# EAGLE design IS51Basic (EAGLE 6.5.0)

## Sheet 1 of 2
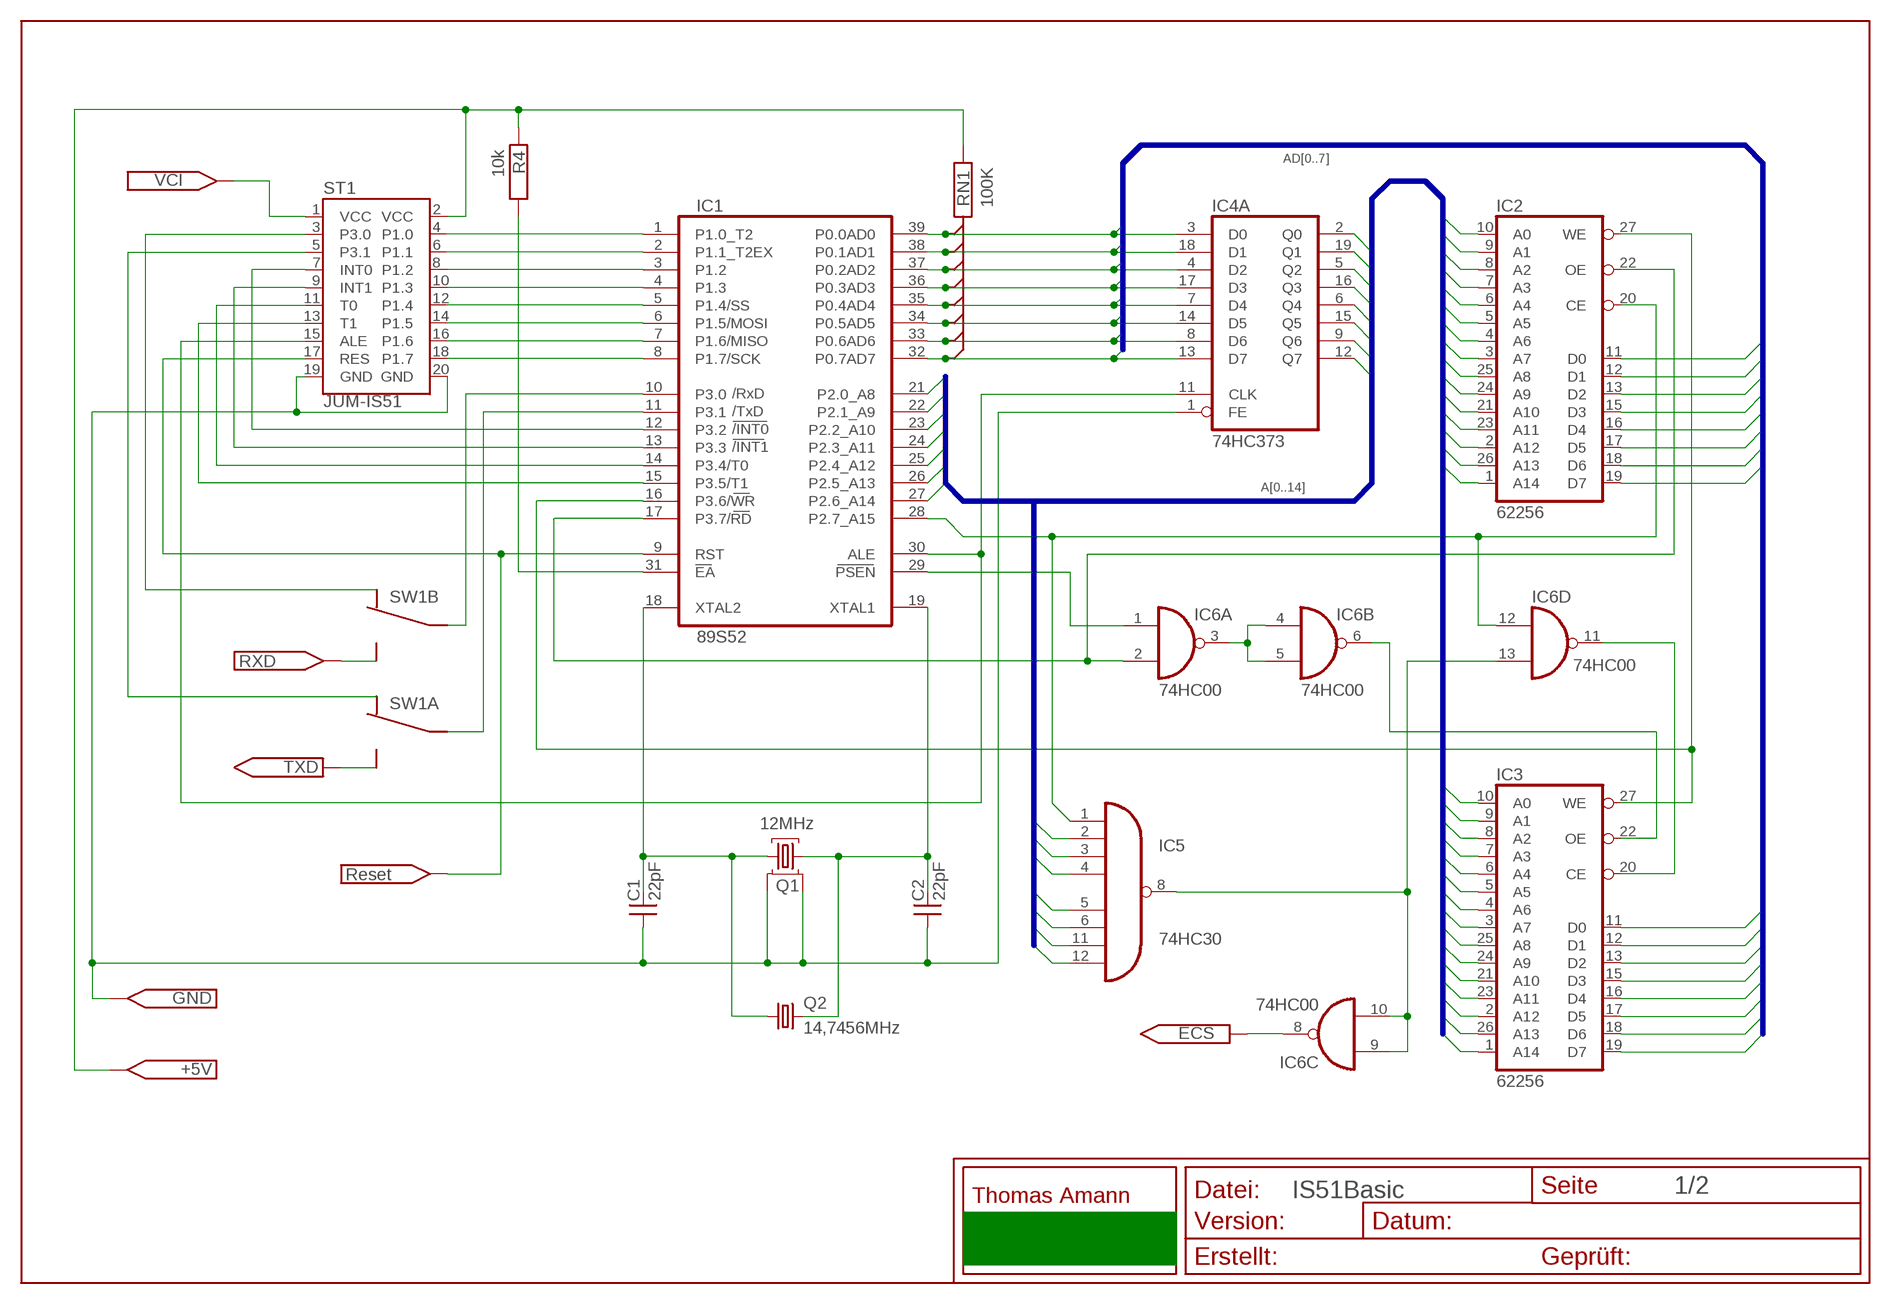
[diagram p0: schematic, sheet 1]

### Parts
C1  22pF  C2_025  [C2_025]
C2  22pF  C2_025  [C2_025]
IC1  89S52  89S8253  [DIL40]
IC2  62256  62256DIL28_SMAL  [DIL28_S]
IC3  62256  [DIL28]
IC4  74HC373  74373_1  [DIL20]
IC5  74HC30  74HC30N  [DIL14]
IC6  74HC00  74HC00N  [DIL14]
Q1  12MHz  QUARZ4  [QCTS406]
Q2  14,7456MHz  CRYSTALHC49S  [HC49/S]
R4  10k  R025A  [R025A]
RN1  100K  RN8_DIL  [RN8_DIL]
ST1  JUM-IS51  [JUM10X2]
SW1  SW2_2XUM  [SW2_2XUM]

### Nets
A0: IC2.10(A0) IC3.10(A0) IC4.2(A:Q0) ; also sheet 2
A1: IC2.9(A1) IC3.9(A1) IC4.19(A:Q1) ; also sheet 2
A2: IC2.8(A2) IC3.8(A2) IC4.5(A:Q2) ; also sheet 2
A3: IC2.7(A3) IC3.7(A3) IC4.16(A:Q3) ; also sheet 2
A4: IC2.6(A4) IC3.6(A4) IC4.6(A:Q4) ; also sheet 2
A5: IC2.5(A5) IC3.5(A5) IC4.15(A:Q5) ; also sheet 2
A6: IC2.4(A6) IC3.4(A6) IC4.9(A:Q6) ; also sheet 2
A7: IC2.3(A7) IC3.3(A7) IC4.12(A:Q7) ; also sheet 2
A8: IC1.21(P2.0_A8) IC2.25(A8) IC3.25(A8) IC5.11(I6) ; also sheet 2
A9: IC1.22(P2.1_A9) IC2.24(A9) IC3.24(A9) IC5.12(I7) ; also sheet 2
A10: IC1.23(P2.2_A10) IC2.21(A10) IC3.21(A10) IC5.6(I5) ; also sheet 2
A11: IC1.24(P2.3_A11) IC2.23(A11) IC3.23(A11) IC5.5(I4) ; also sheet 2
A12: IC1.25(P2.4_A12) IC2.2(A12) IC3.2(A12) IC5.4(I3) ; also sheet 2
A13: IC1.26(P2.5_A13) IC2.26(A13) IC3.26(A13) IC5.3(I2) ; also sheet 2
A14: IC1.27(P2.6_A14) IC2.1(A14) IC3.1(A14) IC5.2(I1) ; also sheet 2
A15: IC1.28(P2.7_A15) IC2.20(CE) IC5.1(I0) IC6.12(D:I0) ; also sheet 2
AD0: IC1.39(P0.0AD0) IC2.11(D0) IC3.11(D0) IC4.3(A:D0) RN1.2 ; also sheet 2
AD1: IC1.38(P0.1AD1) IC2.12(D1) IC3.12(D1) IC4.18(A:D1) RN1.3 ; also sheet 2
AD2: IC1.37(P0.2AD2) IC2.13(D2) IC3.13(D2) IC4.4(A:D2) RN1.4 ; also sheet 2
AD3: IC1.36(P0.3AD3) IC2.15(D3) IC3.15(D3) IC4.17(A:D3) RN1.5 ; also sheet 2
AD4: IC1.35(P0.4AD4) IC2.16(D4) IC3.16(D4) IC4.7(A:D4) RN1.6 ; also sheet 2
AD5: IC1.34(P0.5AD5) IC2.17(D5) IC3.17(D5) IC4.14(A:D5) RN1.7 ; also sheet 2
AD6: IC1.33(P0.6AD6) IC2.18(D6) IC3.18(D6) IC4.8(A:D6) RN1.8 ; also sheet 2
AD7: IC1.32(P0.7AD7) IC2.19(D7) IC3.19(D7) IC4.13(A:D7) RN1.9 ; also sheet 2
ALE: IC1.30(ALE) IC4.11(A:CLK) ST1.15(ALE)
EA: IC1.31(EA) R4.2
ECS: IC6.8(C:O) ; also sheet 2
GND: C1.1 C2.1 IC4.1(A:FE) Q1.2 Q1.4 ST1.19(GND) ST1.20(GND) ; also sheet 2
INT0: IC1.12(P3.2) ST1.7(INT0)
INT1: IC1.13(P3.3) ST1.9(INT1)
N$14: IC3.20(CE) IC6.11(D:O)
N$15: IC5.8(O) IC6.9(C:I0) IC6.10(C:I1) IC6.13(D:I1)
OER: IC3.22(OE) IC6.6(B:O)
OEV: IC6.3(A:O) IC6.4(B:I0) IC6.5(B:I1)
P10: IC1.1(P1.0_T2) ST1.4(P1.0)
P11: IC1.2(P1.1_T2EX) ST1.6(P1.1)
P12: IC1.3(P1.2) ST1.8(P1.2)
P13: IC1.4(P1.3) ST1.10(P1.3)
P14: IC1.5(P1.4/SS) ST1.12(P1.4)
P15: IC1.6(P1.5/MOSI) ST1.14(P1.5)
P16: IC1.7(P1.6/MISO) ST1.16(P1.6)
P17: IC1.8(P1.7/SCK) ST1.18(P1.7)
P30: ST1.3(P3.0) SW1.6
P31: ST1.5(P3.1) SW1.1
PSEN: IC1.29(PSEN) IC6.1(A:I0)
RD: IC1.17(P3.7/RD) IC2.22(OE) IC6.2(A:I1) ; also sheet 2
RES: IC1.9(RST) ST1.17(RES) ; also sheet 2
RXP: IC1.10(P3.0) SW1.5
T0: IC1.14(P3.4/T0) ST1.11(T0)
T1: IC1.15(P3.5/T1) ST1.13(T1)
TXD: SW1.3 ; also sheet 2
TXP: IC1.11(P3.1) SW1.2
VCC: R4.1 RN1.1 ST1.2(VCC) ; also sheet 2
VCI: ST1.1(VCC) ; also sheet 2
WR: IC1.16(P3.6/WR) IC2.27(WE) IC3.27(WE) ; also sheet 2
XT1: C2.2 IC1.19(XTAL1) Q1.3 Q2.2
XT2: C1.2 IC1.18(XTAL2) Q1.1 Q2.1
XYZ: SW1.4 ; also sheet 2

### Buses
A[0..14]
AD[0..7]

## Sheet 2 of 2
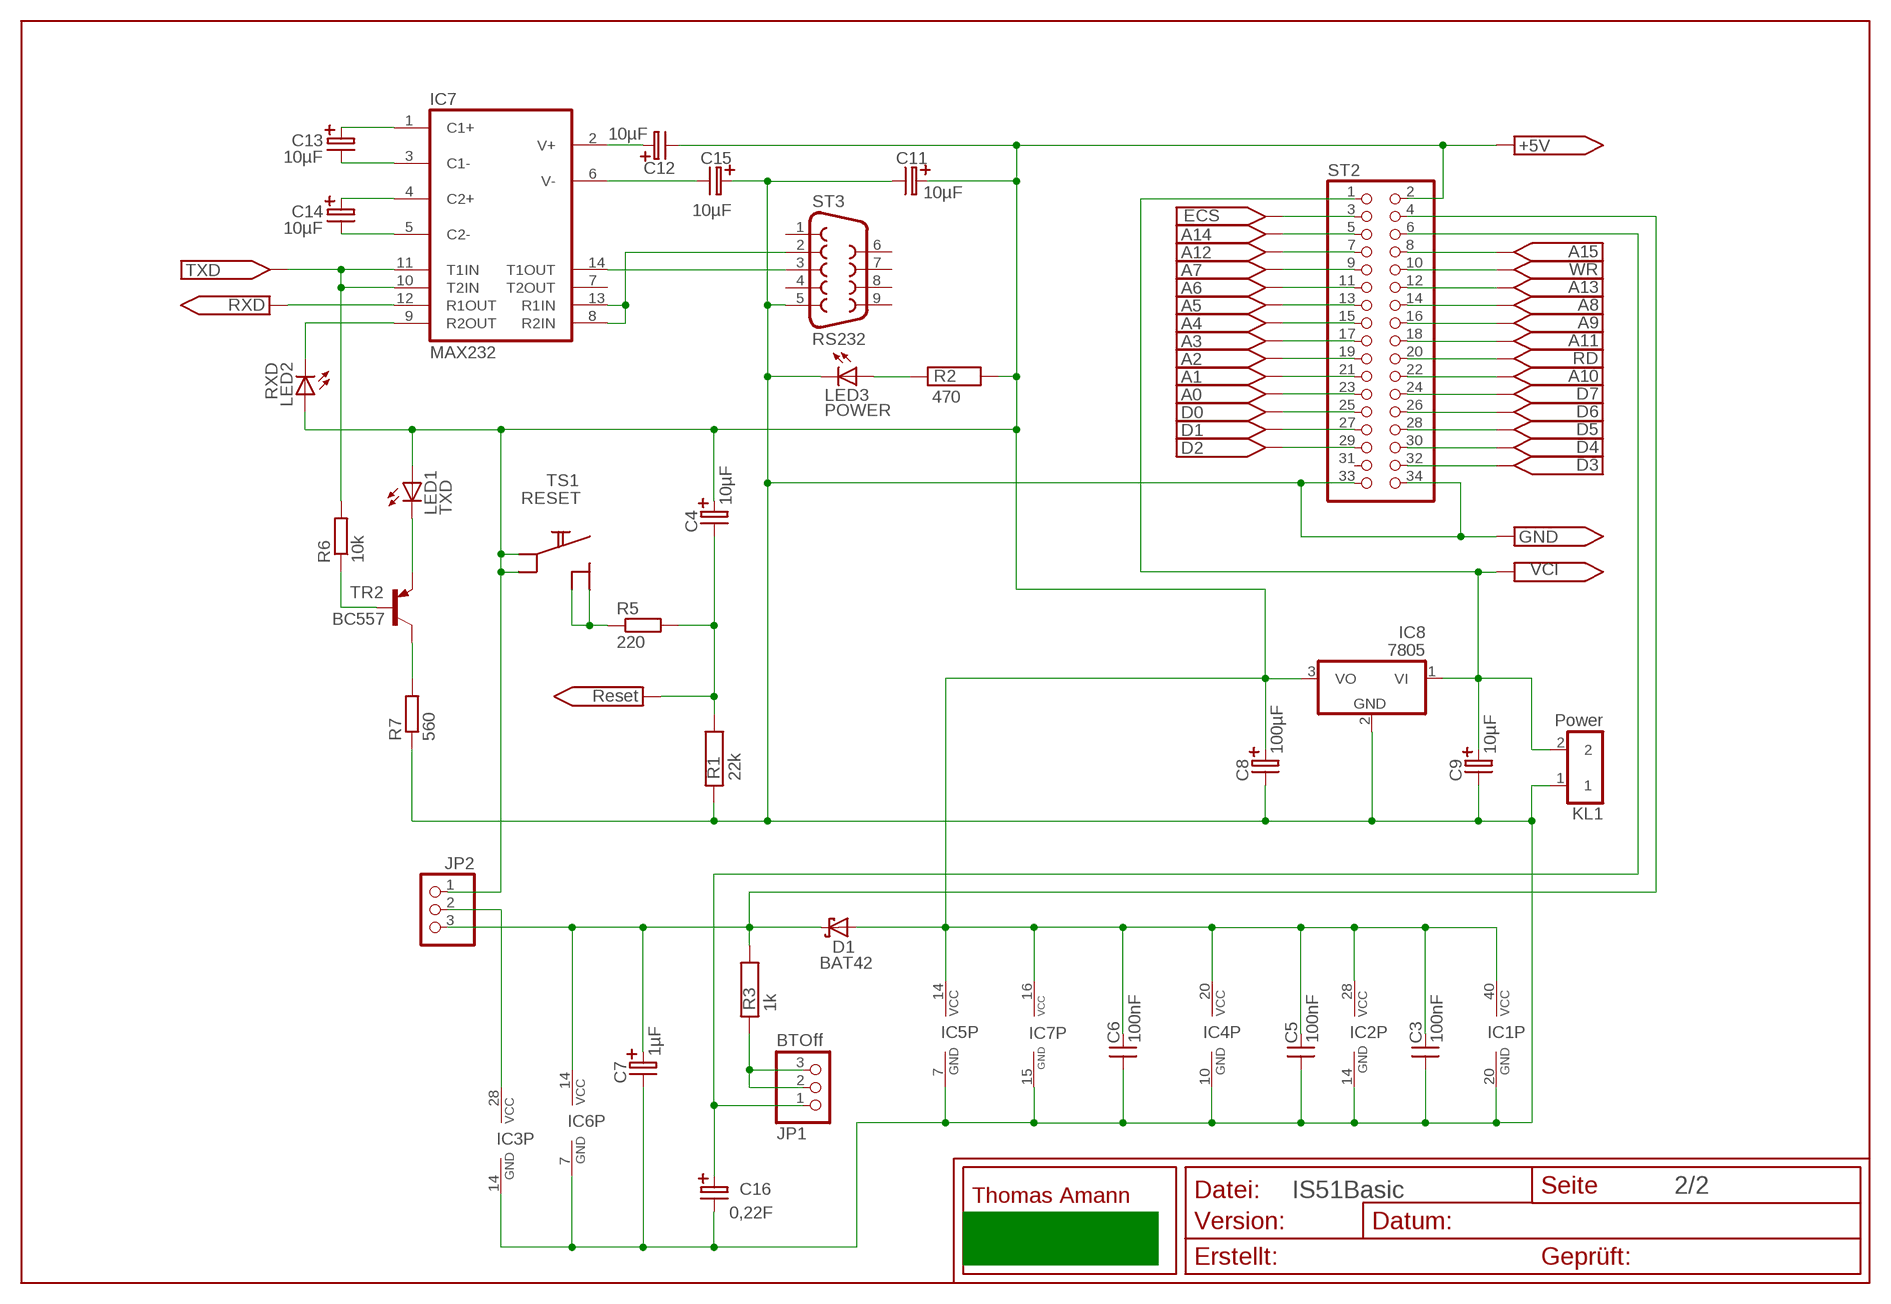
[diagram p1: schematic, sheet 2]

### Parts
C3  100nF  C2_05  [C2_05]
C4  10µF  TELK1_25  [TELK1_25]
C5  100nF  C2_05  [C2_05]
C6  100nF  C2_05  [C2_05]
C7  1µF  TELK1_25  [TELK1_25]
C8  100µF  TELK1_25  [TELK1_25]
C9  10µF  TELK1_25  [TELK1_25]
C11  10µF  TELK1_25  [TELK1_25]
C12  10µF  TELK1_25  [TELK1_25]
C13  10µF  TELK1_25  [TELK1_25]
C14  10µF  TELK1_25  [TELK1_25]
C15  10µF  TELK1_25  [TELK1_25]
C16  0,22F  E50_125R  [E50_125R]
D1  BAT42  [DO35-10]
IC7  MAX232  [DIL16]
IC8  7805  7805TV  [TO220V]
JP1  BTOff  PINHD-1X3  [1X03]
JP2  PINHD-1X3  [1X03]
KL1  Power  KL2_5  [KL2_5]
LED1  TXD  LED3MM  [LED3MM]
LED2  RXD  LED3MM  [LED3MM]
LED3  POWER  LED3MM  [LED3MM]
R1  22k  R025A  [R025A]
R2  470  R025A  [R025A]
R3  1k  R025A  [R025A]
R5  220  R-EU_R1206  [R1206]
R6  10k  R-EU_R1206  [R1206]
R7  560  R-EU_R1206  [R1206]
ST2  PINHD-2X17  [2X17]
ST3  RS232  F09H  [F09H]
TR2  BC557  BC327  [TO92]
TS1  RESET  MTAST  [MTAST]

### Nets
A0: ST2.23 ; also sheet 1
A1: ST2.21 ; also sheet 1
A2: ST2.19 ; also sheet 1
A3: ST2.17 ; also sheet 1
A4: ST2.15 ; also sheet 1
A5: ST2.13 ; also sheet 1
A6: ST2.11 ; also sheet 1
A7: ST2.9 ; also sheet 1
A8: ST2.14 ; also sheet 1
A9: ST2.16 ; also sheet 1
A10: ST2.22 ; also sheet 1
A11: ST2.18 ; also sheet 1
A12: ST2.7 ; also sheet 1
A13: ST2.12 ; also sheet 1
A14: ST2.5 ; also sheet 1
A15: ST2.8 ; also sheet 1
AD0: ST2.25 ; also sheet 1
AD1: ST2.27 ; also sheet 1
AD2: ST2.29 ; also sheet 1
AD3: ST2.32 ; also sheet 1
AD4: ST2.30 ; also sheet 1
AD5: ST2.28 ; also sheet 1
AD6: ST2.26 ; also sheet 1
AD7: ST2.24 ; also sheet 1
ECS: ST2.3 ; also sheet 1
GND: C3.1 C5.1 C6.1 C7.K C8.K C9.K C11.K C15.A C16.K IC1.20(GND) IC2.14(GND) IC3.14(GND) IC4.10(P:GND) IC5.7(GND) IC6.7(P:GND) IC7.15(GND) IC8.2(GND) KL1.1 LED3.K(C) R1.1 R7.1 ST2.33 ST2.34 ST3.5 ; also sheet 1
N$1: C13.K IC7.3(C1-)
N$4: C13.A IC7.1(C1+)
N$6: LED3.A R2.1
N$13: LED1.K(C) TR2.1(E)
N$18: C14.A IC7.4(C2+)
N$19: C14.K IC7.5(C2-)
N$23: R6.1 TR2.2(B)
N$25: R7.2 TR2.3(C)
N$28: IC7.14(T1OUT) ST3.3
N$29: IC7.8(R2IN) IC7.13(R1IN) ST3.2
N$31: C15.K IC7.6(V-)
N$32: C12.A IC7.2(V+)
N$49: R5.1 TS1.3 TS1.4
RD: ST2.20 ; also sheet 1
RES: C4.K R1.2 R5.2 ; also sheet 1
RXL: IC7.9(R2OUT) LED2.K(C)
TXD: IC7.10(T2IN) IC7.11(T1IN) R6.2 ; also sheet 1
VCB: C16.A JP1.1 ST2.6
VCC: C3.2 C4.A C5.2 C6.2 C8.A C11.A C12.K D1.A IC1.40(VCC) IC2.28(VCC) IC4.20(P:VCC) IC5.14(VCC) IC7.16(VCC) IC8.3(VO) JP2.1 LED1.A LED2.A R2.2 ST2.2 TS1.1 TS1.2 ; also sheet 1
VCI: C9.A IC8.1(VI) KL1.2 ST2.1 ; also sheet 1
VCP: C7.A D1.C IC6.14(P:VCC) JP2.3 R3.2 ST2.4
VCR: IC3.28(VCC) JP2.2
VCV: JP1.2 JP1.3 R3.1
WR: ST2.10 ; also sheet 1
XYZ: IC7.12(R1OUT) ; also sheet 1
Unconnected: IC7.7(T2OUT) ST2.31 ST3.1 ST3.4 ST3.6 ST3.7 ST3.8 ST3.9

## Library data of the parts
C1 C2 = RUNDC:C2_025
C3 C5 C6 = RUNDC:C2_05
C4 C7-C9 C11-C15 = RUNDC:TELK1_25
C16 = RUNDC:E50_125R
D1 = diode:BAT42: DIODE
IC1 = IS-51:89S8253: Grundmodel 8051/32 in DIL40 und PLCC44
IC2 = MyMemory:62256: Static-RAM 32k x 8
IC3 = memory:62256
IC4 = IS-51:74373_1: 74373 mit D0-D7 Belegung von oben nach unten
IC5 = 74xx-eu:74*30: 8-input NAND gate
IC6 = 74xx-eu:74*00: Quad 2-input NAND gate
IC7 = maxim:MAX232: RS232 TRANSEIVER
IC8 = linear:78*: Positive VOLTAGE REGULATOR Source: http://cache.national.com/ds/LM/LM78L05.pdf http://www.fairchildsemi.com/ds/LM/LM7805.pdf
JP1 JP2 = pinhead:PINHD-1X3: PIN HEADER
KL1 = TOMLIB:KL2_5
LED1-LED3 = led:LED: LED
Q1 = TOMLIB:QUARZ4
Q2 = crystal:CRYSTAL: CRYSTAL
R1-R4 = RUNDC:R025A
R5-R7 = resistor:R-EU_: RESISTOR, European symbol
RN1 = RUNDC:RN8_DIL
ST1 = IS-51:JUM-IS51: 20pol. Stecker für Erweiterung der IS51
ST2 = pinhead:PINHD-2X17: PIN HEADER
ST3 = con-subd:F09: SUB-D
SW1 = TOMLIB:SW2_2XUM
TR2 = transistor-pnp:BC327: PNP Transistor
TS1 = TOMLIB:MTAST: Einfacher Taster mit zwei paralellen Kontakten

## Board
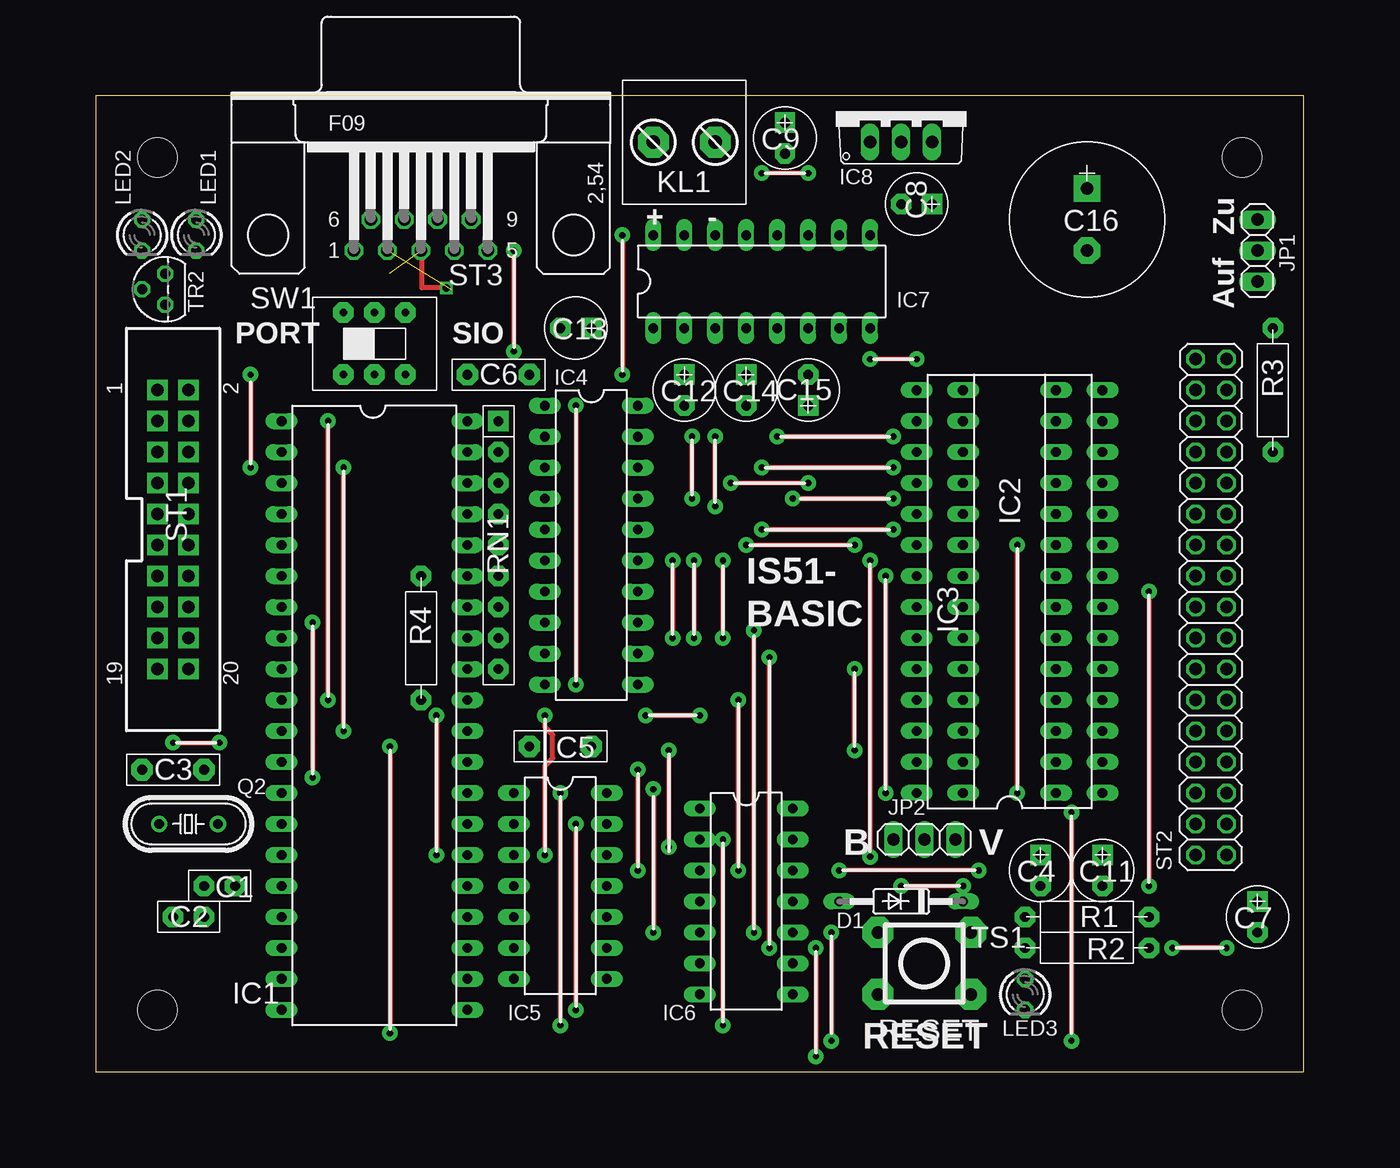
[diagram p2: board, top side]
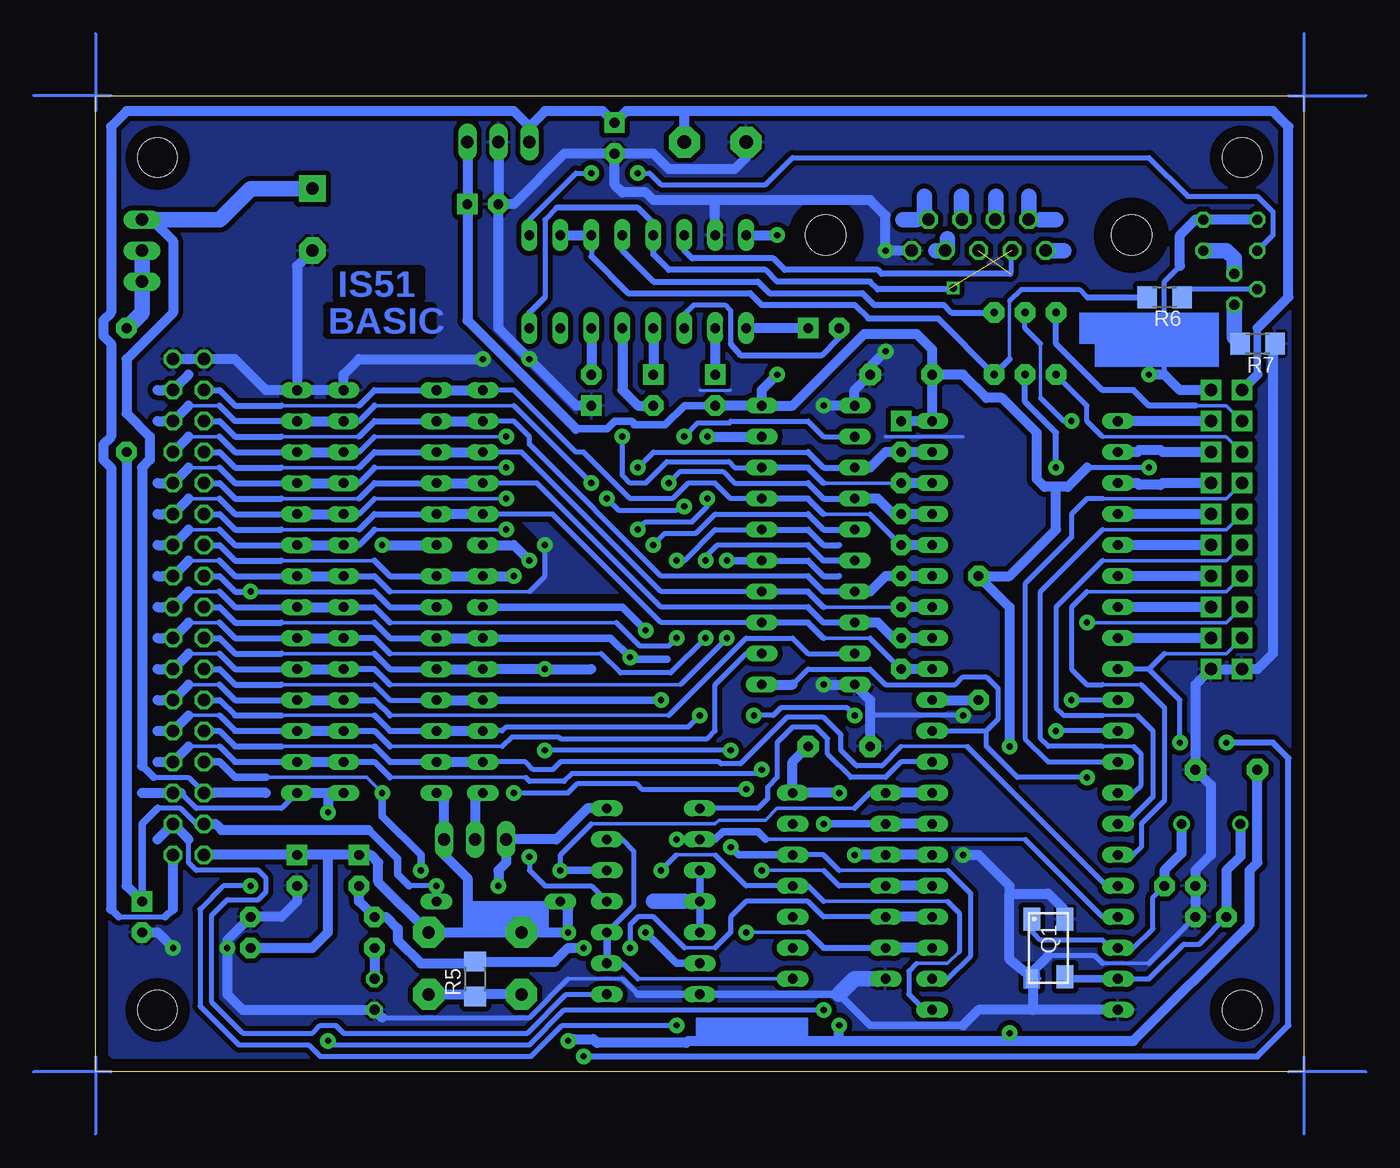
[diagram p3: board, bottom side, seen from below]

Size 99.04 x 80 mm. Coordinates in mm from the lower left corner, seen from the top.
Outline: 0,0 99.04,0 99.04,80 0,80 0,0
Copper layers (1*16): Top 0.035mm / dielectric 1.5mm / Bottom 0.035mm
Design rules "default": minimum track width 10mil, minimum drill 24mil, track to track 8mil, track to pad 8mil, pad to pad 8mil, via to via 8mil, smd to smd 8mil, copper to edge 40mil, drill to drill 8mil, minimum pad ring 10mil, minimum via ring 8mil, stop-mask expansion 4mil, vias tented up to drill 0mil, thermal gap 10mil
Holes 3.2 mm at 5.08,74.93 5.08,5.08 93.98,5.08 93.98,74.93

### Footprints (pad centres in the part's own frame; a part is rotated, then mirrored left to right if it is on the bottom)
C2_025 = drill 0.813 pad 1.676 octagon: 1 -1.27,0; 2 1.27,0
C2_05 = drill 0.813 pad 1.778 octagon: 1 0,0; 2 5.08,0
TELK1_25 = drill 0.813 pad 1.676 square: A 0,0 | drill 0.813 pad 1.676 octagon: K 0,-2.54
E50_125R = drill 1.016 pad 2.184 square: A 0,0 | drill 1.016 pad 2.184 octagon: K 0,-5.08
DO35-10 = drill 0.813 long: A 5.08,0; C -5.08,0
DIL40 = drill 0.813 long: 1 -24.13,-7.62; 2 -21.59,-7.62; 3 -19.05,-7.62; 4 -16.51,-7.62; 5 -13.97,-7.62; 6 -11.43,-7.62; 7 -8.89,-7.62; 8 -6.35,-7.62; 9 -3.81,-7.62; 10 -1.27,-7.62; 11 1.27,-7.62; 12 3.81,-7.62; 13 6.35,-7.62; 14 8.89,-7.62; 15 11.43,-7.62; 16 13.97,-7.62; 17 16.51,-7.62; 18 19.05,-7.62; 19 21.59,-7.62; 20 24.13,-7.62; 21 24.13,7.62; 22 21.59,7.62; 23 19.05,7.62; 24 16.51,7.62; 25 13.97,7.62; 26 11.43,7.62; 27 8.89,7.62; 28 6.35,7.62; 29 3.81,7.62; 30 1.27,7.62; 31 -1.27,7.62; 32 -3.81,7.62; 33 -6.35,7.62; 34 -8.89,7.62; 35 -11.43,7.62; 36 -13.97,7.62; 37 -16.51,7.62; 38 -19.05,7.62; 39 -21.59,7.62; 40 -24.13,7.62; 41 -24.13,-7.62
DIL28_S = drill 0.813 long: 1 -16.51,-3.81; 2 -13.97,-3.81; 3 -11.43,-3.81; 4 -8.89,-3.81; 5 -6.35,-3.81; 6 -3.81,-3.81; 7 -1.27,-3.81; 8 1.27,-3.81; 9 3.81,-3.81; 10 6.35,-3.81; 11 8.89,-3.81; 12 11.43,-3.81; 13 13.97,-3.81; 14 16.51,-3.81; 15 16.51,3.81; 16 13.97,3.81; 17 11.43,3.81; 18 8.89,3.81; 19 6.35,3.81; 20 3.81,3.81; 21 1.27,3.81; 22 -1.27,3.81; 23 -3.81,3.81; 24 -6.35,3.81; 25 -8.89,3.81; 26 -11.43,3.81; 27 -13.97,3.81; 28 -16.51,3.81
DIL28 = drill 0.813 long: 1 -16.51,-7.62; 2 -13.97,-7.62; 3 -11.43,-7.62; 4 -8.89,-7.62; 5 -6.35,-7.62; 6 -3.81,-7.62; 7 -1.27,-7.62; 8 1.27,-7.62; 9 3.81,-7.62; 10 6.35,-7.62; 11 8.89,-7.62; 12 11.43,-7.62; 13 13.97,-7.62; 14 16.51,-7.62; 15 16.51,7.62; 16 13.97,7.62; 17 11.43,7.62; 18 8.89,7.62; 19 6.35,7.62; 20 3.81,7.62; 21 1.27,7.62; 22 -1.27,7.62; 23 -3.81,7.62; 24 -6.35,7.62; 25 -8.89,7.62; 26 -11.43,7.62; 27 -13.97,7.62; 28 -16.51,7.62
DIL20 = drill 0.813 long: 1 -11.43,-3.81; 2 -8.89,-3.81; 3 -6.35,-3.81; 4 -3.81,-3.81; 5 -1.27,-3.81; 6 1.27,-3.81; 7 3.81,-3.81; 8 6.35,-3.81; 9 8.89,-3.81; 10 11.43,-3.81; 11 11.43,3.81; 12 8.89,3.81; 13 6.35,3.81; 14 3.81,3.81; 15 1.27,3.81; 16 -1.27,3.81; 17 -3.81,3.81; 18 -6.35,3.81; 19 -8.89,3.81; 20 -11.43,3.81; 21 -11.43,-3.81
DIL14 = drill 0.813 long: 1 -7.62,-3.81; 2 -5.08,-3.81; 3 -2.54,-3.81; 4 0,-3.81; 5 2.54,-3.81; 6 5.08,-3.81; 7 7.62,-3.81; 8 7.62,3.81; 9 5.08,3.81; 10 2.54,3.81; 11 0,3.81; 12 -2.54,3.81; 13 -5.08,3.81; 14 -7.62,3.81
DIL16 = drill 0.813 long: 1 -8.89,-3.81; 2 -6.35,-3.81; 3 -3.81,-3.81; 4 -1.27,-3.81; 5 1.27,-3.81; 6 3.81,-3.81; 7 6.35,-3.81; 8 8.89,-3.81; 9 8.89,3.81; 10 6.35,3.81; 11 3.81,3.81; 12 1.27,3.81; 13 -1.27,3.81; 14 -3.81,3.81; 15 -6.35,3.81; 16 -8.89,3.81
TO220V = drill 1.016 long: 1 -2.54,-2.54; 2 0,-2.54; 3 2.54,-2.54
1X03 = drill 1.016 long: 1 -2.54,0; 2 0,0; 3 2.54,0
KL2_5 = drill 1.1 pad 2.54 octagon: 1 0,0; 2 5.08,0
LED3MM = drill 0.813 octagon: A -1.27,0; K 1.27,0
QCTS406 = smd 1.9 x 1.4: 1 -2.362,-1.362; 3 2.362,1.362; 4 -2.362,1.362 | smd 1.524 x 1.016: 2 2.518,-1.362
HC49/S = drill 0.813: 1 -2.413,0; 2 2.413,0
R025A = drill 0.813 pad 1.676 octagon: 1 -5.08,0; 2 5.08,0
R1206 = smd 1.6 x 1.803: 1 -1.422,0; 2 1.422,0
RN8_DIL = drill 0.813 pad 1.676 square: 1 0,0 | drill 0.813 pad 1.676 octagon: 2 2.54,0; 3 5.08,0; 4 7.62,0; 5 10.16,0; 6 12.7,0; 7 15.24,0; 8 17.78,0; 9 20.32,0
JUM10X2 = drill 1.016 pad 1.676 square: 1 0,0; 2 0,2.54; 3 2.54,0; 4 2.54,2.54; 5 5.08,0; 6 5.08,2.54; 7 7.62,0; 8 7.62,2.54; 9 10.16,0; 10 10.16,2.54; 11 12.7,0; 12 12.7,2.54; 13 15.24,0; 14 15.24,2.54; 15 17.78,0; 16 17.78,2.54; 17 20.32,0; 18 20.32,2.54; 19 22.86,0; 20 22.86,2.54
2X17 = drill 1.016 octagon: 1 -20.32,-1.27; 2 -20.32,1.27; 3 -17.78,-1.27; 4 -17.78,1.27; 5 -15.24,-1.27; 6 -15.24,1.27; 7 -12.7,-1.27; 8 -12.7,1.27; 9 -10.16,-1.27; 10 -10.16,1.27; 11 -7.62,-1.27; 12 -7.62,1.27; 13 -5.08,-1.27; 14 -5.08,1.27; 15 -2.54,-1.27; 16 -2.54,1.27; 17 0,-1.27; 18 0,1.27; 19 2.54,-1.27; 20 2.54,1.27; 21 5.08,-1.27; 22 5.08,1.27; 23 7.62,-1.27; 24 7.62,1.27; 25 10.16,-1.27; 26 10.16,1.27; 27 12.7,-1.27; 28 12.7,1.27; 29 15.24,-1.27; 30 15.24,1.27; 31 17.78,-1.27; 32 17.78,1.27; 33 20.32,-1.27; 34 20.32,1.27
F09H = drill 1.016 octagon: 1 -5.486,-1.27; 2 -2.743,-1.27; 3 0,-1.27; 4 2.743,-1.27; 5 5.486,-1.27; 6 -4.115,1.27; 7 -1.372,1.27; 8 1.372,1.27; 9 4.115,1.27 | hole 3.302: -12.522,0; 12.522,0
SW2_2XUM = drill 0.61 pad 1.676 octagon: 1 -2.54,-2.54; 2 0,-2.54; 3 2.54,-2.54; 4 2.54,2.54; 5 0,2.54; 6 -2.54,2.54
TO92 = drill 0.813 octagon: 1 1.27,0; 2 0,1.905; 3 -1.27,0
MTAST = drill 1.016 pad 2.54 octagon: 1 -3.81,2.54; 2 3.81,2.54; 3 -3.81,-2.54; 4 3.81,-2.54

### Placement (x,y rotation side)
C1  10.16,15.24 0 top
C2  7.62,12.7 180 top
C3  8.89,24.77 180 top
C4  77.47,17.78 0 top
C5  35.56,26.67 0 top
C6  35.56,57.15 180 top
C7  95.25,13.97 0 top
C8  68.58,71.12 270 top
C9  56.52,77.79 0 top
C11  82.55,17.78 0 top
C12  48.26,57.15 0 top
C13  40.64,60.96 270 top
C14  53.34,57.15 0 top
C15  58.42,54.61 180 top
C16  81.28,72.39 0 top
D1  66.04,13.97 180 top
IC1  22.86,29.21 270 top
IC2  74.93,39.37 90 top
IC3  74.93,39.37 90 top
IC4  40.64,43.18 270 top
IC5  38.1,15.24 270 top
IC6  53.34,13.97 270 top
IC7  54.61,64.77 0 top
IC8  66.04,78.74 0 top
JP1  95.25,67.31 270 top
JP2  67.94,19.05 180 top
KL1  45.72,76.2 0 top
LED1  8.26,68.58 270 top
LED2  3.81,68.58 270 top
LED3  76.2,6.35 270 top
Q1  20.95,10.16 270 bottom
Q2  7.62,20.32 180 top
R1  81.28,12.7 180 top
R2  81.28,10.16 0 top
R3  96.52,55.88 270 top
R4  26.67,35.56 270 top
R5  67.94,7.62 90 bottom
R6  11.43,63.5 180 bottom
R7  3.81,59.69 180 bottom
RN1  33.02,53.34 270 top
ST1  5.08,55.88 270 top
ST2  91.44,38.1 90 top
ST3  26.67,68.58 0 top
SW1  22.86,59.69 0 top
TR2  5.71,64.14 90 top
TS1  67.94,8.89 0 top

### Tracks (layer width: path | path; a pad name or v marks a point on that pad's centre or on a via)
A0  (via drill 0.5 pad 1.27)
  Top 0.406: v65.41,46.99 v57.15,46.99 | v50.8,46.35 v50.8,52.07
  Bottom 0.305: 91.44,46.99 88.9,46.99 | 76.2,46.99 v65.41,46.99
  Bottom 0.406: IC2.10 77.47,45.72 76.2,46.99 | v57.15,46.99 56.2,46.04 51.44,46.04 51.12,46.35 v50.8,46.35 | v50.8,52.07 49.69,53.18 47.15,53.18 arc-90 46.99,53.34 40.64,53.34 39.37,52.07 IC4.2
  Bottom 0.508: 88.9,46.99 87.63,45.72 IC3.10
  Bottom 0.813: ST2.23 91.44,46.99 | IC3.10 IC2.10
A1  (via drill 0.5 pad 1.27)
  Top 0.406: v65.41,44.45 v54.61,44.45 | v48.9,46.99 v48.9,52.07
  Bottom 0.305: 91.44,44.45 88.9,44.45 | 76.2,44.45 v65.41,44.45
  Bottom 0.406: v54.61,44.45 53.98,45.09 50.16,45.09 48.9,46.35 v48.9,46.99
  Bottom 0.508: 88.9,44.45 87.63,43.18 IC3.9 | IC2.9 77.47,43.18 76.2,44.45
  Bottom 0.813: ST2.21 91.44,44.45 | IC3.9 IC2.9 | v48.9,52.07 IC4.19
A2  (via drill 0.5 pad 1.27)
  Top 0.406: v62.23,43.18 v53.34,43.18
  Bottom 0.305: 91.44,41.91 88.9,41.91 | 74.93,39.37 63.5,39.37
  Bottom 0.406: 63.5,39.37 62.23,40.64 v62.23,43.18 | v53.34,43.18 52.39,44.13 49.85,44.13 48.26,45.72 40.64,45.72
  Bottom 0.508: 88.9,41.91 87.63,40.64 IC3.8 | IC2.8 76.2,40.64 74.93,39.37 | 40.64,45.72 39.37,44.45 IC4.5
  Bottom 0.813: ST2.19 91.44,41.91 | IC3.8 IC2.8
  pour Bottom (isolate 0.406): 56.2,39.21 62.07,45.09 64.14,45.09 62.23,43.18 62.23,40.64 63.34,39.21
A3  (via drill 0.5 pad 1.27)
  Top 0.406: v51.44,35.56 v51.44,41.91
  Bottom 0.305: 91.44,39.37 88.9,39.37 | 74.93,36.83 56.36,36.83
  Bottom 0.406: 56.36,36.83 54.45,34.92 52.07,34.92 v51.44,35.56 | v51.44,41.91 50.8,41.91 48.26,44.45 IC4.16
  Bottom 0.508: 88.9,39.37 87.63,38.1 IC3.7 | IC2.7 76.2,38.1 74.93,36.83 | IC4.16 40.64,44.45 39.37,43.18 38.1,43.18
  Bottom 0.813: ST2.17 91.44,39.37 | IC3.7 IC2.7
A4  (via drill 0.5 pad 1.27)
  Top 0.406: v49.05,41.91 v49.05,35.56
  Bottom 0.305: 91.44,36.83 88.9,36.83 | 57.63,34.29 74.93,34.29
  Bottom 0.406: 40.64,43.18 48.1,43.18 49.05,42.23 v49.05,41.91 | v49.05,35.56 51.91,32.7 56.04,32.7 57.63,34.29
  Bottom 0.508: 88.9,36.83 87.63,35.56 IC3.6 | IC4.6 39.37,41.91 40.64,43.18 | 74.93,34.29 76.2,35.56 IC2.6
  Bottom 0.813: ST2.15 91.44,36.83 | IC3.6 IC2.6
A5  (via drill 0.5 pad 1.27)
  Top 0.406: v47.31,41.91 v47.31,35.56
  Bottom 0.305: 91.44,34.29 88.9,34.29 | 51.12,31.75 74.93,31.75
  Bottom 0.406: v47.31,35.56 51.12,31.75
  Bottom 0.508: 88.9,34.29 87.63,33.02 IC3.5 | 74.93,31.75 76.2,33.02 IC2.5 | IC4.15 40.64,41.91 39.37,40.64 38.1,40.64
  Bottom 0.61: IC4.15 v47.31,41.91
  Bottom 0.813: ST2.13 91.44,34.29 | IC3.5 IC2.5
A6
  Bottom 0.305: 91.44,31.75 88.9,31.75 | 74.93,29.21 52.07,29.21
  Bottom 0.406: 52.07,29.21 45.72,35.56 41.91,35.56 40.64,34.29 IC4.9
  Bottom 0.508: 88.9,31.75 87.63,30.48 IC3.4 | IC2.4 76.2,30.48 74.93,29.21
  Bottom 0.813: ST2.11 91.44,31.75 | IC3.4 IC2.4
A7
  Bottom 0.305: 91.44,29.21 88.9,29.21 | 74.93,26.67 65.72,26.67
  Bottom 0.406: 65.72,26.67 64.93,27.46 61.12,27.46 60.96,27.3 48.9,27.3 48.26,27.94 48.26,31.75 45.72,34.29 IC4.12
  Bottom 0.508: 88.9,29.21 87.63,27.94 IC3.3 | IC2.3 76.2,27.94 74.93,26.67
  Bottom 0.813: ST2.9 91.44,29.21 | IC3.3 IC2.3
A8  (via drill 0.5 pad 1.27)
  Top 0.406: v52.7,16.51 v52.7,30.48
  Bottom 0.305: 83.82,31.75 76.2,31.75 | 48.26,17.78 51.44,17.78 | 39.37,13.97 29.21,13.97 | 28.26,9.84 29.21,8.89 31.75,8.89
  Bottom 0.406: 76.2,31.75 74.93,30.48 IC2.25 | IC1.21 31.11,5.08 32.38,6.35 32.38,8.26 31.75,8.89 | 39.37,13.97 40.64,15.24 IC5.11 45.72,15.24 48.26,17.78 | 51.44,17.78 v52.7,16.51 | 29.21,13.97 28.26,13.02 28.26,9.84
  Bottom 0.508: ST2.14 88.9,33.02 87.63,31.75 83.82,31.75
  Bottom 0.61: v52.7,30.48 IC3.25
  Bottom 0.813: IC2.25 IC3.25
A9  (via drill 0.5 pad 1.27)
  Top 0.406: v46.99,18.41 v46.99,26.35 | v62.23,26.35 v62.23,33.02
  Bottom 0.305: 83.82,34.29 76.2,34.29 | 29.21,16.51 38.1,16.51
  Bottom 0.406: IC1.22 29.21,7.62 27.3,9.53 27.3,14.61 29.21,16.51 | 38.1,16.51 39.37,17.78 IC5.12 | v46.99,26.35 v62.23,26.35
  Bottom 0.508: ST2.16 88.9,35.56 87.63,34.29 83.82,34.29 | 76.2,34.29 74.93,33.02 IC2.24
  Bottom 0.61: IC5.12 46.35,17.78 v46.99,18.41
  Bottom 0.813: IC2.24 IC3.24 v62.23,33.02 58.42,33.02
A10  (via drill 0.5 pad 1.27)
  Top 0.406: v64.77,40.64 v64.77,22.86 | v45.72,23.18 v45.72,11.43
  Bottom 0.305: 83.82,41.91 76.2,41.91 | v45.72,11.43 40.64,11.43
  Bottom 0.406: v64.77,22.86 60.33,22.86 59.53,23.65 54.77,23.65 54.29,23.18 v45.72,23.18
  Bottom 0.508: ST2.22 88.9,43.18 87.63,41.91 83.82,41.91 | 76.2,41.91 74.93,40.64 IC2.21 | 40.64,11.43 39.37,10.16 IC5.6
  Bottom 0.813: IC2.21 IC3.21 v64.77,40.64 | IC1.23 IC5.6
A11  (via drill 0.5 pad 1.27)
  Top 0.406: v55.24,10.16 v55.24,33.97
  Bottom 0.305: 83.82,36.83 76.2,36.83 | 48.26,10.16 50.8,10.16
  Bottom 0.406: IC5.5 39.37,12.7 40.64,13.97 45.72,13.97 46.99,12.7 46.99,11.43 48.26,10.16 | 50.8,10.16 53.34,12.7 54.61,12.7 55.24,12.06 v55.24,10.16
  Bottom 0.508: ST2.18 88.9,38.1 87.63,36.83 83.82,36.83 | 76.2,36.83 74.93,35.56 IC2.23
  Bottom 0.61: v55.24,33.97 56.83,35.56 IC3.23
  Bottom 0.813: IC2.23 IC3.23 | IC1.24 IC5.5
A12  (via drill 0.5 pad 1.27)
  Top 0.406: v44.45,16.51 v44.45,24.77
  Bottom 0.305: 91.44,26.67 88.9,26.67 | 39.37,16.51 v44.45,16.51 | 63.82,24.13 74.93,24.13
  Bottom 0.406: IC5.4 38.1,15.24 39.37,16.51 | v44.45,24.77 44.77,24.45 60.01,24.45 60.64,23.81 63.5,23.81 63.82,24.13
  Bottom 0.508: 88.9,26.67 87.63,25.4 IC3.2 | IC2.2 76.2,25.4 74.93,24.13
  Bottom 0.813: ST2.7 91.44,26.67 | IC3.2 IC2.2 | IC1.25 IC5.4
A13  (via drill 0.5 pad 1.27)
  Top 0.406: v36.83,17.78 36.83,25.08 37.47,25.72 37.47,27.62 36.83,28.26 v36.83,29.21 | v45.09,29.21 v49.53,29.21
  Bottom 0.305: 83.82,29.21 76.2,29.21
  Bottom 0.406: v36.83,29.21 37.47,29.84 42.86,29.84 43.5,29.21 v45.09,29.21 | v49.53,29.21 50.48,28.26 65.41,28.26 65.72,27.94 IC3.26
  Bottom 0.508: ST2.12 88.9,30.48 87.63,29.21 83.82,29.21 | 76.2,29.21 74.93,27.94 IC2.26
  Bottom 0.813: IC2.26 IC3.26 | IC1.26 IC5.3 v36.83,17.78
A14  (via drill 0.5 pad 1.27)
  Top 0.406: v80.01,21.27 v80.01,2.54 | v39.37,5.08 v39.37,20.32
  Bottom 0.406: IC3.1 83.82,21.59 90.81,21.59 92.08,22.86 | v80.01,2.54 79.69,2.22 63.5,2.22 60.64,5.08 v39.37,5.08
  Bottom 0.61: v39.37,20.32 IC5.2
  Bottom 0.813: IC1.27 IC5.2 | 92.08,22.86 ST2.5 | IC3.1 80.01,22.86 | IC2.1 80.01,22.86 | 80.01,22.86 v80.01,21.27
A15  (via drill 0.5 pad 1.27)
  Top 0.406: v75.56,22.86 v75.56,43.18 | v72.39,16.51 v60.96,16.51
  Bottom 0.305: 85.09,24.13 76.83,24.13 v75.56,22.86 | 36.83,21.59 43.18,21.59 44.13,20.64 47.94,20.64 48.26,20.32 58.42,20.32
  Bottom 0.406: IC5.1 35.56,22.86 36.83,21.59 | 58.42,20.32 60.96,17.78 v60.96,16.51
  Bottom 0.61: ST2.8 88.9,25.4 87.63,24.13 85.09,24.13 | v60.96,16.51 IC6.12 | v75.56,22.86 75.56,20.95 72.39,17.78 v72.39,16.51
  Bottom 0.813: IC1.28 IC5.1 | v75.56,43.18 IC2.20
AD0  (via drill 0.5 pad 1.27)
  Top 0.406: v65.41,49.53 v54.61,49.53
  Bottom 0.305: 91.44,49.53 88.9,49.53 | 76.2,49.53 v65.41,49.53
  Bottom 0.406: v54.61,49.53 53.34,50.8 40.64,50.8
  Bottom 0.508: 88.9,49.53 87.63,48.26 IC3.11 | IC2.11 77.47,48.26 76.2,49.53 | 40.64,50.8 39.37,49.53 IC4.3
  Bottom 0.813: ST2.25 91.44,49.53 | IC3.11 IC2.11 | IC1.39 RN1.2 34.29,50.8 35.56,49.53 IC4.3
AD1  (via drill 0.5 pad 1.27)
  Top 0.406: v65.41,52.07 v55.88,52.07
  Bottom 0.305: 91.44,52.07 88.9,52.07 | RN1.3 39.37,48.26 | 76.2,52.07 v65.41,52.07
  Bottom 0.406: IC2.12 77.47,50.8 76.2,52.07 | IC4.18 46.67,49.53 47.15,50.01 52.23,50.01 53.98,48.26 55.24,48.26 55.88,48.9 v55.88,52.07
  Bottom 0.508: 88.9,52.07 87.63,50.8 IC3.12 | 39.37,48.26 40.64,49.53 IC4.18
  Bottom 0.813: ST2.27 91.44,52.07 | IC3.12 IC2.12 | IC1.38 RN1.3
AD2  (via drill 0.5 pad 1.27)
  Top 0.406: v58.42,48.26 v52.07,48.26
  Bottom 0.305: 88.9,54.61 91.44,54.61 | 76.2,54.61 64.77,54.61
  Bottom 0.406: 64.77,54.61 v58.42,48.26 | v52.07,48.26 51.12,49.21 47.62,49.21 46.67,48.26 40.64,48.26
  Bottom 0.508: IC3.13 87.63,53.34 88.9,54.61 | IC2.13 77.47,53.34 76.2,54.61 | 40.64,48.26 39.37,46.99 IC4.4
  Bottom 0.813: 91.44,54.61 ST2.29 | IC3.13 IC2.13 | IC1.37 RN1.4 33.66,45.72 34.92,46.99 IC4.4
AD3
  Bottom 0.305: 83.82,54.61 77.47,54.61 | 35.56,45.72 39.37,45.72
  Bottom 0.406: RN1.5 35.56,45.72 | IC4.17 46.99,46.99 48.26,48.26 50.48,48.26 51.75,46.99 55.24,46.99 59.05,50.8 59.69,50.8 64.77,55.88 IC3.15
  Bottom 0.508: ST2.32 88.9,55.88 87.63,54.61 83.82,54.61 | 77.47,54.61 76.2,55.88 IC2.15 | 39.37,45.72 40.64,46.99 IC4.17
  Bottom 0.813: IC2.15 IC3.15 | IC1.36 RN1.5
AD4
  Bottom 0.305: 83.82,52.07 77.47,52.07
  Bottom 0.406: 40.64,40.64 52.7,40.64 63.5,51.44 63.5,52.07 64.77,53.34 IC3.16
  Bottom 0.508: ST2.30 88.9,53.34 87.63,52.07 83.82,52.07 | 77.47,52.07 76.2,53.34 IC2.16 | IC4.7 39.37,39.37 40.64,40.64
  Bottom 0.813: IC2.16 IC3.16 | IC1.35 RN1.6 34.29,40.64 35.56,39.37 IC4.7
AD5
  Bottom 0.305: 83.82,49.53 77.47,49.53 | RN1.7 39.37,38.1
  Bottom 0.406: IC4.14 52.7,39.37 64.14,50.8 IC3.17
  Bottom 0.508: ST2.28 88.9,50.8 87.63,49.53 83.82,49.53 | 77.47,49.53 76.2,50.8 IC2.17 | 39.37,38.1 40.64,39.37 IC4.14
  Bottom 0.813: IC2.17 IC3.17 | IC1.34 RN1.7
AD6
  Bottom 0.305: 83.82,46.99 77.47,46.99
  Bottom 0.406: 40.64,38.1 52.7,38.1 62.87,48.26 IC3.18
  Bottom 0.508: ST2.26 88.9,48.26 87.63,46.99 83.82,46.99 | 77.47,46.99 76.2,48.26 IC2.18 | IC4.8 39.37,36.83 40.64,38.1
  Bottom 0.813: IC2.18 IC3.18 | IC1.33 RN1.8 33.66,35.56 34.92,36.83 IC4.8
AD7
  Bottom 0.305: 83.82,44.45 77.47,44.45 | 35.56,35.56 39.37,35.56
  Bottom 0.406: RN1.9 35.56,35.56 | IC4.13 52.7,36.83 61.59,45.72 IC3.19
  Bottom 0.508: ST2.24 88.9,45.72 87.63,44.45 83.82,44.45 | 77.47,44.45 76.2,45.72 IC2.19 | 39.37,35.56 40.64,36.83 IC4.13
  Bottom 0.813: IC1.32 RN1.9 | IC3.19 IC2.19
ALE  (via drill 0.5 pad 1.27)
  Top 0.406: v17.78,36.83 v17.78,24.13
  Bottom 0.305: ST1.15 6.35,36.83 v17.78,36.83
  Bottom 0.406: v17.78,24.13 23.5,24.13 26.04,26.67 26.04,27.94 | IC1.30 26.04,27.94 | 41.91,31.75 40.64,33.02 35.56,33.02 34.29,31.75 28.57,31.75 27.94,32.38 26.04,32.38 25.08,31.43 25.08,28.89 26.04,27.94
  Bottom 0.813: IC4.11 41.91,31.75
EA
  Bottom 0.813: IC1.31 R4.2
ECS
  Bottom 0.406: IC6.8 60.48,6.35 63.66,3.17 78.74,3.17 79.38,3.81 80.64,3.81 81.28,3.17 87,3.17 89.53,5.71 89.53,12.86 88.27,14.13 85.72,14.13 85.09,14.76 85.09,15.88 85.72,16.51 90.81,16.51 91.44,17.14 91.44,19.05
  Bottom 0.813: 91.44,19.05 ST2.3
GND  (via drill 0.5 pad 1.27)
  Top 0.406: v39.37,54.61 v39.37,31.75 | v67.31,58.42 v63.5,58.42 | v27.94,29.21 v27.94,17.78 | v92.71,10.16 v88.27,10.16 | v34.29,59.05 v34.29,67.31
  Bottom 0.254: 22.23,7.62 22.32,6.89 Q1.2 21.61,7.64 22.54,7.94 | Q1.4 19.59,13.24 | 49.53,55.88 46.99,55.88
  Bottom 0.305: 60.33,7.62 55.88,7.62 | 12.7,8.89 16.51,8.89 | 34.29,52.07 27.94,52.07
  Bottom 0.406: R7.1 2.54,59.69 | 75.56,4.45 63.5,4.45 60.33,7.62 | 55.88,7.62 54.61,6.35 | 16.51,8.89 17.14,9.53 20.95,9.53 | 12.7,8.89 C2.1 | v27.94,29.21 35.56,29.21
  Bottom 0.61: 54.61,6.35 IC6.7 38.1,6.35 35.56,3.81 27.94,3.81
  Bottom 0.813: IC3.14 IC2.14 78.74,57.15 77.47,58.42 v67.31,58.42 | IC3.14 85.09,55.88 87.63,58.42 ST2.34 ST2.33 | IC1.20 22.23,5.08 | 22.23,5.08 26.67,5.08 27.94,3.81 | 22.23,7.62 22.23,5.08 | 24.13,14.61 24.13,9.21 22.54,7.94 20.95,9.53 | 24.13,14.61 20.95,14.61 19.59,13.24 | v39.37,54.61 IC4.1 36.83,55.88 C6.1 35.56,57.78 v34.29,59.05 | v39.37,31.75 IC4.10 35.56,30.48 35.56,29.21 C5.1 | ST3.5 v34.29,67.31 34.29,70.17 35.56,71.44 48.26,71.44 | 48.26,71.44 53.34,71.44 53.98,72.07 55.88,72.07 56.52,72.71 C9.K | C9.K 53.34,75.25 52.07,73.98 46.67,73.98 45.72,74.93 KL1.1 | IC7.15 48.26,71.44 | IC8.2 C8.K | C9.K 60.64,75.25 64.77,71.12 C8.K | C15.A 59.69,54.61 v63.5,58.42 66.04,60.96 C8.K | 2.54,59.69 2.54,34.29 3.81,33.02 ST1.19 ST1.20 8.89,31.75 C3.1 7.62,23.5 7.62,17.78 8.89,16.51 C1.1 C2.1 | C16.K 82.55,66.04 IC3.14 | C11.K 82.55,13.97 83.82,12.7 R1.1 88.27,10.79 v88.27,10.16 88.27,6.35 87,5.08 LED3.K 75.56,4.45 | v27.94,17.78 26.67,17.78 24.13,15.24 24.13,14.61 | C7.K 93.98,11.43 v92.71,10.16
  Bottom 1.27: IC5.7 36.83,7.62 38.1,6.35
  pour Bottom (isolate 0.406): 0,77.47 2.54,80.01 96.52,80.01 99.06,77.47 99.06,2.54 96.52,0 2.54,0 0,2.54
INT0
  Bottom 0.305: ST1.7 6.35,46.99 16.51,46.99
  Bottom 0.406: 16.51,46.99 17.78,46.99 19.05,45.72 19.05,43.81 22.86,40.01 22.86,27.3 20.95,25.4 IC1.12
INT1
  Bottom 0.305: 13.97,26.67 16.51,26.67 | 16.51,44.45 6.35,44.45 ST1.9
  Bottom 0.406: IC1.13 13.97,22.86 13.34,23.5 13.34,26.04 13.97,26.67 | 16.51,26.67 20.95,26.67 21.59,27.3 21.59,39.37 16.51,44.45
N$1
  Bottom 0.406: IC7.3 50.8,62.07 50.01,62.87 47.47,62.87 46.99,62.39 46.99,59.69
  Bottom 0.508: 46.99,59.69 46.2,58.74 39.53,58.74 38.1,60.17 C13.K
N$2
  Bottom 0.254: 0,85.09 0,78.74
N$3
  Bottom 0.254: 1.27,80.01 -5.08,80.01
N$4
  Bottom 0.813: C13.A IC7.1
N$5
  Bottom 0.254: 99.06,85.09 99.06,78.74
N$6
  Bottom 0.813: R2.1 LED3.A
N$7
  Bottom 1.27: 31.11,70.48 31.11,71.75
N$8
  Bottom 0.254: 97.79,80.01 104.14,80.01
N$9
  Bottom 0.254: -5.08,0 1.27,0
N$10
  Bottom 0.254: 0,1.27 0,-5.08
N$11
  Bottom 0.254: 97.79,0 104.14,0
N$12
  Bottom 0.254: 99.06,1.27 99.06,-5.08
N$13
  Bottom 1.27: TR2.1 5.71,66.67 6.35,67.31 LED1.K
N$14  (via drill 0.5 pad 1.27)
  Top 0.406: v63.5,41.91 v63.5,17.62
  Bottom 0.406: v63.5,17.62 63.5,16.51 62.23,15.24 58.42,15.24 IC6.11
  Bottom 0.813: IC3.20 64.77,43.18 v63.5,41.91
N$15
  Bottom 0.305: 54.61,7.62 IC5.8
  Bottom 0.406: IC6.10 54.93,13.65 54.93,18.1 55.88,19.05 IC6.13 | IC6.9 55.88,8.89 54.61,7.62
  Bottom 0.61: IC6.10 IC6.9
N$16
  Bottom 1.27: 28.1,70.48 28.1,71.75
N$17
  Bottom 1.27: 25.24,70.48 25.24,71.75
N$18
  Bottom 0.813: IC7.4 C14.A
N$19
  Bottom 0.813: IC7.5 55.88,55.88 54.61,54.61 C14.K
N$20
  Bottom 1.27: 22.54,69.85 22.54,71.75
N$21
  Bottom 1.27: 20.95,67.31 19.68,67.31
N$22
  Bottom 1.27: 29.21,68.26 29.21,67.31 30.16,67.31
N$23
  Bottom 0.254: 9.4,64.14 R6.1
  Bottom 0.406: TR2.2 9.4,64.14
N$24
  Bottom 1.27: 20.32,69.85 21.59,69.85
N$25
  Bottom 0.254: 5.71,60.2 R7.2
  Bottom 1.27: TR2.3 5.71,60.2
N$26
  Bottom 1.27: 32.86,69.85 31.75,69.85
N$27
  Bottom 0.813: 91.44,57.15 92.39,56.2
N$28  (1 unrouted)
  Bottom 0.508: 24.07,65.41 34.61,65.41 34.92,65.72 42.55,65.72 43.5,66.67 50.16,66.67 50.8,67.31 IC7.14
N$29  (2 unrouted)
  Bottom 0.406: 61.28,70.8 62.23,69.85 62.23,63.5 | 63.5,62.23 IC7.8
  Bottom 0.508: 61.28,70.8 54.61,70.8 53.34,69.53 IC7.13 53.34,66.99 52.07,65.72 44.13,65.72 43.18,64.77 35.56,64.77 34.92,64.14 29.15,64.14 | 62.23,63.5 63.5,62.23
N$30
  Bottom 0.813: 93.98,55.88 93.5,55.88
N$31
  Bottom 0.813: IC7.6 C15.K
N$32
  Bottom 0.813: IC7.2 C12.A
N$33
  Bottom 0.813: 93.98,53.34 93.5,53.34
N$34
  Bottom 0.813: 93.98,48.26 93.34,48.26
N$35
  Bottom 0.813: 93.98,45.72 93.5,45.72
N$36
  Bottom 0.813: 93.98,43.18 93.5,43.18
N$37
  Bottom 0.813: 93.98,40.64 93.5,40.64
N$38
  Bottom 0.813: 93.98,38.1 93.5,38.1
N$39
  Bottom 0.813: 93.98,35.56 93.5,35.56
N$40
  Bottom 0.813: 93.98,33.02 93.5,33.02
N$41
  Bottom 0.813: 93.98,30.48 93.5,30.48
N$42
  Bottom 0.813: 93.98,27.94 93.5,27.94
N$43
  Bottom 0.813: 93.98,25.4 93.19,25.4
N$44
  Bottom 0.813: 95.25,22.86 93.34,22.86
N$45
  Bottom 0.813: 93.98,19.05 93.34,19.68
N$46
  Bottom 0.813: 85.09,22.86 89.38,22.86
N$47
  Bottom 0.61: 54.77,33.81 52.23,33.81
N$48
  Bottom 1.27: 53.34,13.97 50.8,13.97
N$49
  Bottom 0.813: TS1.3 67.82,6.35 R5.1 68.07,6.35 TS1.4
N$50
  Bottom 0.406: 24,65.5 24,67.25
N$51  (via drill 0.6)
  Top 0.406: v28.75,64.25 26.75,64.25 26.75,67.25
OER  (via drill 0.5 pad 1.27)
  Top 0.406: v53.98,11.43 v53.98,36.2
  Bottom 0.61: IC6.6 51.44,8.89 v53.98,11.43 | v53.98,36.2 55.88,38.1 IC3.22
OEV
  Bottom 0.61: IC6.3 IC6.4 IC6.5
P10
  Bottom 0.813: ST1.4 IC1.1
P11
  Bottom 0.813: ST1.6 11.59,50.8 11.75,50.96 13.49,50.96 13.65,50.8 IC1.2
P12
  Bottom 0.813: ST1.8 11.59,48.26 11.75,48.1 13.49,48.1 13.65,48.26 IC1.3
P13
  Bottom 0.813: ST1.10 IC1.4
P14
  Bottom 0.813: ST1.12 IC1.5
P15
  Bottom 0.813: ST1.14 IC1.6
P16
  Bottom 0.813: ST1.16 IC1.7
P17
  Bottom 0.813: ST1.18 IC1.8
P30
  Bottom 0.305: ST1.3 6.35,54.61 8.89,54.61
  Bottom 0.508: 8.89,54.61 12.7,54.61 13.97,55.88 16.51,55.88 20.32,59.69 SW1.6
P31
  Bottom 0.305: ST1.5 6.35,52.07 16.51,52.07
  Bottom 0.406: 16.51,52.07 17.78,53.34 17.78,54.61 SW1.1
PSEN
  Bottom 0.406: IC1.29 33.02,25.4 34.29,24.13 37.15,24.13 39.05,26.04 39.05,27.3 40.01,28.26 41.91,28.26 43.18,26.99 43.18,24.13 43.97,23.34 43.97,22.38 44.77,21.59 IC6.1
RD  (via drill 0.5 pad 1.27)
  Top 0.406: v86.36,39.37 v86.36,15.24 | v51.44,3.81 v51.44,19.05
  Bottom 0.305: 22.86,19.05 44.13,19.05
  Bottom 0.406: IC1.17 16.51,12.7 22.86,19.05 | v86.36,15.24 88.58,15.24 90.49,13.34 90.49,5.4 87.31,2.22 81.6,2.22 80.64,1.27 63.34,1.27 60.8,3.81 v51.44,3.81 | v86.36,39.37 76.2,39.37
  Bottom 0.508: ST2.20 88.9,40.64 87.63,39.37 v86.36,39.37 | 76.2,39.37 74.93,38.1 IC2.22
  Bottom 0.61: 44.13,19.05 44.77,19.68 47.62,19.68 48.26,19.05 IC6.2 v51.44,19.05
RES  (via drill 0.5 pad 1.27)
  Top 0.406: v59.05,10.16 v59.05,1.27 | v6.35,26.99 v10.16,26.99
  Bottom 0.305: ST1.17 6.35,34.29 11.43,34.29
  Bottom 0.406: 11.43,34.29 12.7,33.02 | 12.7,33.02 IC1.9 | v10.16,26.99 10.16,30.48 12.7,33.02
  Bottom 0.508: v59.05,1.27 3.81,1.27 1.27,3.81 1.27,25.72 2.54,26.99 v6.35,26.99
  Bottom 0.813: C4.K 77.47,13.97 R1.2 75.25,12.7 74.3,11.75 74.3,10.79 72.39,8.89 68.07,8.89 R5.2 61.47,9.02 60.33,10.16 v59.05,10.16
RXL  (via drill 0.5 pad 1.27)
  Top 0.406: v58.42,73.66 v54.61,73.66
  Bottom 0.406: IC7.9 63.5,69.85 59.69,73.66 v58.42,73.66 | v54.61,73.66 53.66,73.66 52.7,72.71 44.13,72.71 41.91,74.93 12.7,74.93 9.53,71.75 3.81,71.75 2.54,70.48 2.54,68.58 LED2.K
RXP  (via drill 0.5 pad 1.27)
  Top 0.406: v19.05,30.48 v19.05,53.34
  Bottom 0.305: 21.59,55.24 21.59,59.69
  Bottom 0.406: IC1.10 v19.05,30.48 | v19.05,53.34 19.68,53.34 21.59,55.24 | 21.59,59.69 22.86,60.96 SW1.5
T0
  Bottom 0.305: ST1.11 6.35,41.91 16.51,41.91 | 16.51,29.21 13.65,29.21
  Bottom 0.406: 16.51,41.91 20.32,38.1 20.32,29.84 19.68,29.21 16.51,29.21 | 13.65,29.21 12.38,27.94 12.38,22.54 14.61,20.32 IC1.14
T1
  Bottom 0.305: ST1.13 6.35,39.37 17.78,39.37 | 16.51,31.75 13.34,31.75
  Bottom 0.406: 17.78,39.37 19.05,38.1 19.05,33.02 17.78,31.75 16.51,31.75 | 13.34,31.75 11.43,29.84 11.43,22.23 13.34,20.32 13.34,18.41 13.97,17.78 IC1.15
TXD
  Bottom 0.305: 24.13,58.42 24.13,63.18
  Bottom 0.406: 24.13,63.18 23.18,64.14 18.41,64.14 17.78,63.5 | IC7.11 58.42,66.83
  Bottom 0.508: 24.13,58.42 SW1.3 30,61.75 35.72,61.75 36.83,62.87 44.45,62.87 45.4,63.82 55.4,63.82 58.42,66.83 | 17.78,63.5 R6.2
  Bottom 0.813: IC7.10 IC7.11
TXP  (via drill 0.5 pad 1.27)
  Top 0.406: v20.32,27.94 v20.32,49.53
  Bottom 0.406: IC1.11 v20.32,27.94
  Bottom 0.508: v20.32,49.53 20.32,52.39 22.86,54.93 SW1.2
VCB
  Bottom 0.406: 94.3,24.13 91.44,24.13 ST2.6
  Bottom 0.61: 95.25,25.08 94.3,24.13
  Bottom 0.813: 94.46,69.85 92.71,68.1 92.71,62.23 96.52,58.42 96.52,53.98 94.61,52.07 94.61,50.16 95.25,49.53 95.25,25.08
  Bottom 1.27: C16.A 86.36,72.39 88.9,69.85 94.46,69.85 JP1.1
VCC  (via drill 0.5 pad 1.27)
  Top 0.406: v38.1,3.81 v38.1,22.86 | v60.33,11.43 v60.33,2.54 | v12.7,57.15 v12.7,49.53 | v24.13,26.67 v24.13,3.17 | v43.18,68.58 v43.18,57.15
  Bottom 0.406: 11.43,57.15 11.43,64.77 10.16,66.04 | 8.89,69.85 LED1.A | v12.7,49.53 17.78,49.53 | v24.13,3.17 24.13,2.54
  Bottom 0.61: 59.69,52.7 57.15,52.7 56.52,53.34 55.24,53.34 arc90 54.93,53.02 52.39,53.02 50.8,54.61 C12.K
  Bottom 0.813: LED2.A LED1.A | ST1.2 10.16,55.88 11.43,57.15 v12.7,57.15 | 10.16,66.04 10.16,68.58 8.89,69.85 | IC8.3 C8.A 68.58,61.59 59.69,52.7 | C5.2 41.91,25.4 IC5.14 v38.1,22.86 | IC4.20 C12.K | C6.2 IC1.40 RN1.1 | 20.32,47.94 20.32,44.45 24.13,40.64 R4.1 24.13,38.1 v24.13,26.67 | IC4.20 41.91,54.61 36.04,60.48 31.75,60.48 30.48,59.21 C6.2 | 80.01,17.78 C4.A 76.52,17.78 75.88,17.14 75.88,15.56 TS1.2 68.58,11.43 | 80.01,17.78 C11.A ST2.2 | R2.2 81.28,10.16 80.01,11.43 80.01,17.78 | 68.58,11.43 TS1.1 v60.33,11.43 60.33,13.34 D1.A | 38.1,2.54 v38.1,3.81 | v60.33,2.54 60.01,2.54 59.85,2.7 58.26,2.7 57.94,2.38 50.64,2.38 50.48,2.54 38.1,2.54 | 38.1,2.54 24.13,2.54 13.97,2.54 4.45,12.06 4.45,16.51 3.81,17.14 C3.2 | IC2.28 70.48,22.23 JP2.1 70.48,17.78 68.58,15.88 68.58,11.43 | 17.78,49.53 19.37,47.94 20.32,47.94 | 20.32,47.94 21.27,47.94 21.91,48.58 21.91,52.39 24.77,55.24 26.04,55.24 27.94,57.15 C6.2 | IC7.16 v43.18,68.58 | v43.18,57.15 44.45,55.88 IC4.20
VCI
  Bottom 0.406: 97.16,12.7 93.34,12.7
  Bottom 0.61: 3.81,57.15 3.81,60.96 | 97.79,13.34 97.16,12.7 | 93.34,12.7 92.71,13.34
  Bottom 0.813: ST1.1 3.81,57.15 | 3.81,60.96 1.27,63.5 1.27,77.47 2.54,78.74 50.8,78.74 | 50.8,78.74 55.56,78.74 C9.A 57.47,78.74 62.23,78.74 63.5,77.47 | IC8.1 63.5,77.47 | 63.5,77.47 64.77,78.74 96.52,78.74 97.79,77.47 97.79,62.23 98.42,61.59 98.42,60.33 97.79,59.69 97.79,52.07 98.42,51.44 98.42,50.16 97.79,49.53 97.79,13.34 | 92.71,13.34 ST2.1 | KL1.2 50.8,78.74
VCP  (via drill 0.5 pad 1.27)
  Top 0.406: v66.04,15.24 v71.12,15.24
  Bottom 0.406: ST2.4 90.81,20.32 92.08,21.59 93.98,21.59 | v71.12,15.24 73.34,15.24
  Bottom 0.61: 76.68,19.84 74.3,17.46 74.3,16.19 73.34,15.24 | 93.98,21.59 95.25,20.32 C7.A
  Bottom 0.813: R3.2 96.52,15.24 C7.A | ST2.4 89.22,20.32 88.74,19.84 76.68,19.84 | IC6.14 58.74,21.59 61.28,19.05 JP2.3 65.41,17.14 66.04,16.51 v66.04,15.24 | D1.C v71.12,15.24
VCR
  Bottom 0.813: IC3.28 67.94,22.23 JP2.2
VCV
  Bottom 1.27: JP1.2 JP1.3 95.25,62.23 R3.1
WR
  Bottom 0.305: 83.82,26.67 76.2,26.67 | 27.62,26.67 33.02,26.67
  Bottom 0.406: IC1.16 16.19,15.24 27.62,26.67 | IC3.27 63.82,25.4 63.18,24.77 61.59,24.77 60.96,25.4 47.94,25.4 47.78,25.24 46.2,25.24 42.39,29.05 39.37,29.05 37.94,27.62 37.94,26.35 36.67,25.08 34.61,25.08 33.02,26.67
  Bottom 0.508: ST2.10 88.9,27.94 87.63,26.67 83.82,26.67 | 76.2,26.67 74.93,25.4 IC2.27
  Bottom 0.813: IC2.27 IC3.27
XT1
  Bottom 0.406: 19.59,7.62 Q1.3 | IC1.19 12.7,7.62 9.84,10.48 8.57,10.48 C2.2
  Bottom 0.61: IC1.19 19.59,7.62
  Bottom 0.813: Q2.2 5.21,17.65 6.35,16.51 C2.2
XT2
  Bottom 0.406: Q1.1 22.23,12.43 22.23,11.43 21.59,10.79 16.51,10.79 15.88,10.16 IC1.18 13.97,10.16 12.38,11.75 12.38,14.29 C1.2
  Bottom 0.813: Q2.1 10.03,17.91 11.43,16.51 C1.2
XYZ
  Bottom 0.406: 55.88,67.31 IC7.12
  Bottom 0.508: 55.88,67.31 53.34,64.77 44.77,64.77 43.81,63.82 36.2,63.82 35.24,62.87 29.53,62.87 28.89,62.23 SW1.4
(copper drawn outside any net)
  shapes: Bottom area x4, Bottom circle x6

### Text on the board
Bottom: IS51 | BASIC
tPlace: + | - | Zu | Auf | PORT | SIO | IS51- | BASIC | B | V | RESET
